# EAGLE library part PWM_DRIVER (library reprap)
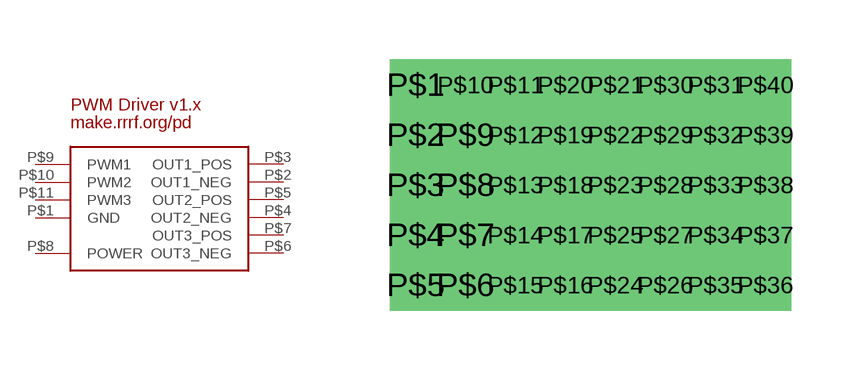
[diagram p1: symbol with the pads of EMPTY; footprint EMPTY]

Designator prefix -

## PWM_DRIVER  [EMPTY]
P$1  GND
P$2  OUT1_NEG
P$3  OUT1_POS
P$4  OUT2_NEG
P$5  OUT2_POS
P$6  OUT3_NEG
P$7  OUT3_POS
P$8  POWER
P$9  PWM1
P$10  PWM2
P$11  PWM3

## Footprint EMPTY (pad centres in mm)
drill 0.8 square: P$1 -1.27,5.08; P$2 -1.27,3.81; P$3 -1.27,2.54; P$4 -1.27,1.27; P$5 -1.27,0; P$6 0,0; P$7 0,1.27; P$8 0,2.54; P$9 0,3.81; P$10 0,5.08; P$11 1.27,5.08; P$12 1.27,3.81; P$13 1.27,2.54; P$14 1.27,1.27; P$15 1.27,0; P$16 2.54,0; P$17 2.54,1.27; P$18 2.54,2.54; P$19 2.54,3.81; P$20 2.54,5.08; P$21 3.81,5.08; P$22 3.81,3.81; P$23 3.81,2.54; P$24 3.81,0; P$25 3.81,1.27; P$26 5.08,0; P$27 5.08,1.27; P$28 5.08,2.54; P$29 5.08,3.81; P$30 5.08,5.08; P$31 6.35,5.08; P$32 6.35,3.81; P$33 6.35,2.54; P$34 6.35,1.27; P$35 6.35,0; P$36 7.62,0; P$37 7.62,1.27; P$38 7.62,2.54; P$39 7.62,3.81; P$40 7.62,5.08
